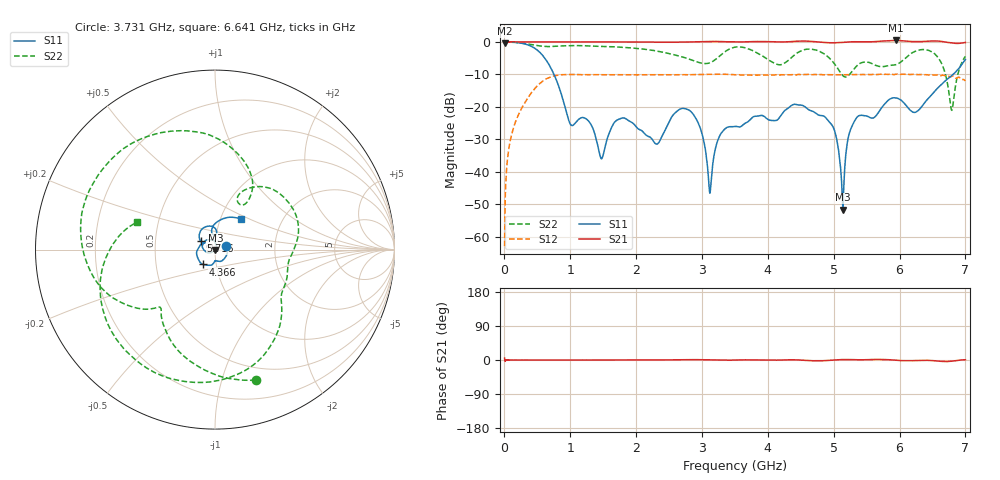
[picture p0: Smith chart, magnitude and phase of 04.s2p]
!Keysight Technologies,N5232A,MY52221221,A.10.65.11
!Date: Wednesday, October 16, 2024 11:52:27
!Correction: S11(Full 2 Port(1,4))
!S41(Full 2 Port(1,4))
!S14(Full 2 Port(1,4))
!S44(Full 2 Port(1,4))
!S2P File: Measurements: S11, S41, S14, S44:
# Hz S  RI  R 50
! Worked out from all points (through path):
!   4000 points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, 2.05 MHz to 7 GHz, reference 50 ohm
!   highest |S21| = 0.44 dB at 5.945 GHz (marker M1); lowest = -0.5 dB at 2.05 MHz (marker M2)
!   lowest |S11| = -51.7 dB at 5.14 GHz (marker M3), VSWR 1.01, Z = 50.2 - j0.181 ohm
!   |S11| at or under -10 dB: 751 MHz to 6.816 GHz (6.065 GHz wide, 160 % of centre)
!   |S22| runs from -21.1 to 0.0 dB; largest |S21 - S12| = 1.3
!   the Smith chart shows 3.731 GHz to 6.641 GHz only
!   S11 on the Smith chart (normalised r, x): 3.731 GHz: 1.13, +0.04; 4.366 GHz: 0.86, -0.14; 5.716 GHz: 0.85, +0.08; 6.641 GHz: 1.25, +0.45
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2049925  -0.9694 0.1504  0.9432 0.0828  0.000138 0.000696  -0.9779 0.0975
1.805423e8  -0.0365 0.9778  0.9998 -0.000118  0.0602 0.0198  -0.8147 0.5443
3.415354e8  0.8925 0.1655  0.9998 -0.000891  0.0872 -0.0979  -0.4297 0.8302
4.867792e8  0.2811 -0.7089  0.9999 -0.00155  -0.0806 -0.1877  -0.0492 0.8797
6.320229e8  -0.4593 -0.258  0.9991 -0.00187  -0.2683 0.0105  0.2717 0.805
1.16925e9  0.0316 0.06  0.9976 -0.00023  0.1622 -0.2665  0.8442 -0.2243
1.687228e9  0.06 0.000665  0.9969 -0.00191  -0.0313 0.3092  -0.1298 -0.8272
2.3347e9  -0.0017 0.0273  0.9912 0.000313  -0.2836 -0.1278  -0.6382 0.3224
2.815929e9  0.0759 -0.0425  0.997 0.0146  0.2958 0.1013  0.1166 0.5243
3.122166e9  0.00203 -0.00426  1.014 0.00823  -0.0504 -0.3121  0.3139 0.359
3.5019e9  -0.0486 0.0109  0.9968 -0.00185  -0.1228 0.2861  0.7896 -0.2546
3.73114e9  0.0601 0.0188  1.007 0.00808  0.2768 0.1327  0.2262 -0.7272
4.366363e9  -0.0665 -0.0824  1.012 0.00946  -0.2481 0.1895  -0.4938 -0.3071
4.66735e9  -0.0822 0.0262  1.015 -0.0341  0.2808 0.1364  -0.6114 0.4659
5.13983e9  0.00185 -0.00181  0.9814 0.021  -0.2847 -0.1259  0.1643 0.252
5.715555e9  -0.0798 0.0471  1.025 0.0265  0.2974 -0.1101  0.4108 -0.064
5.83455e9  -0.0848 0.0954  1.044 0.0136  0.1239 -0.2899  0.4002 -0.16
5.944795e9  -0.0444 0.1296  1.052 -0.0105  -0.1093 -0.2983  0.3708 -0.2467
6.315779e9  -0.0175 0.0928  1.01 -0.0165  -0.0598 0.3079  -0.183 -0.7324
6.641265e9  0.1432 0.1706  1.013 -0.0636  0.2566 -0.1633  -0.4323 0.1535
6.793509e9  0.2901 -0.0821  0.9573 -0.0526  -0.0375 -0.2922  -0.0879 -0.00535
7e9  -0.4455 -0.2994  0.9775 0.0111  -0.2459 0.05  -0.5968 -0.0363
